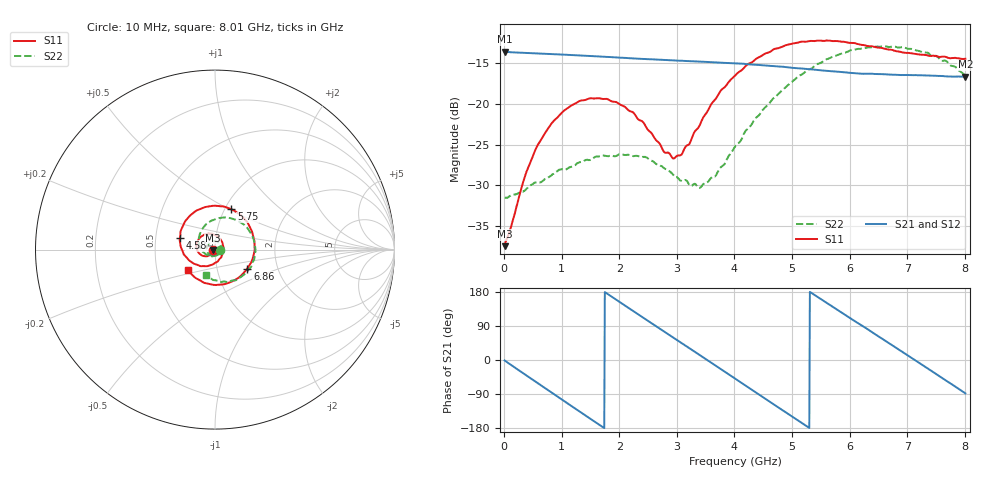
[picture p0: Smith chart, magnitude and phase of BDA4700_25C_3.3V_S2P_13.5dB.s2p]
!Agilent Technologies,E5071B,MY42404982,A.09.10
!Date: Mon Oct 20 18:08:42 2025
!Data & Calibration Information:
!Freq	S11:SOLT2(ON)	S21:SOLT2(ON)	S12:SOLT2(ON)	S22:SOLT2(ON)
# Hz S RI R 50
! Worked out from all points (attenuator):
!   801 points, 10 MHz to 8.01 GHz, reference 50 ohm
!   highest |S21| = -13.60 dB at 10 MHz (marker M1); lowest = -16.7 dB at 8.01 GHz (marker M2)
!   lowest |S11| = -37.5 dB at 10 MHz (marker M3), VSWR 1.03, Z = 48.7 - j0.143 ohm
!   |S11| at or under -10 dB: start of sweep to end of sweep
!   |S22| runs from -31.6 to -12.9 dB; largest |S21 - S12| = 0.0025
!   S11 on the Smith chart (normalised r, x): 10 MHz: 0.97, -0.00; 4.58 GHz: 0.67, +0.09; 5.75 GHz: 1.07, +0.51; 6.86 GHz: 1.40, -0.31; 8.01 GHz: 0.72, -0.17
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1e7  -0.0133 -0.00147  0.2088 -0.00449  0.2087 -0.00475  0.0266 -0.000994
3.6e8  -0.0242 -0.0262  0.1622 -0.1262  0.1622 -0.1262  0.0221 -0.0194
5.8e8  -0.0417 -0.0364  0.1 -0.1777  0.0999 -0.1777  0.0135 -0.03
8.7e8  -0.0716 -0.0333  -0.00207 -0.2016  -0.00192 -0.2017  -0.00896 -0.0364
1.35e9  -0.104 0.0145  -0.1513 -0.1275  -0.1513 -0.1276  -0.0414 -0.0147
1.97e9  -0.0563 0.0846  -0.1769 0.0758  -0.1771 0.0757  -0.0307 0.0373
2.25e9  -0.013 0.087  -0.1182 0.1486  -0.1183 0.1488  -0.00834 0.047
2.68e9  0.0402 0.0419  0.0159 0.1861  0.0155 0.1859  0.0255 0.0334
2.97e9  0.0458 -0.00926  0.1031 0.1529  0.1029 0.1526  0.0342 0.0107
3.09e9  0.0392 -0.0299  0.1329 0.127  0.1317 0.1276  0.0335 -0.000585
3.4e9  0.000208 -0.0741  0.1771 0.04  0.1774 0.0401  0.0185 -0.0242
3.67e9  -0.0542 -0.0918  0.1739 -0.0449  0.174 -0.0453  -0.00593 -0.0357
4.01e9  -0.1317 -0.0691  0.1166 -0.1337  0.1168 -0.1335  -0.0456 -0.0298
4.58e9  -0.1951 0.0658  -0.0492 -0.1643  -0.0489 -0.1645  -0.0896 0.0412
4.94e9  -0.1577 0.1693  -0.1338 -0.1006  -0.1335 -0.1015  -0.0752 0.1076
5.35e9  -0.0447 0.2389  -0.1621 0.012  -0.1621 0.0111  -0.00633 0.1655
5.75e9  0.0915 0.2249  -0.1138 0.1096  -0.1135 0.1097  0.0935 0.1738
6.23e9  0.204 0.1053  0.0021 0.1528  0.00422 0.1528  0.1967 0.0947
6.68e9  0.2094 -0.0504  0.1077 0.1062  0.108 0.1061  0.2218 -0.0275
6.86e9  0.1801 -0.1062  0.1341 0.0682  0.1344 0.0673  0.2075 -0.0774
7.45e9  0.00646 -0.1975  0.1264 -0.0785  0.1265 -0.0788  0.0845 -0.1763
8.01e9  -0.1493 -0.1159  0.0049 -0.1465  0.00538 -0.1466  -0.0496 -0.1409
